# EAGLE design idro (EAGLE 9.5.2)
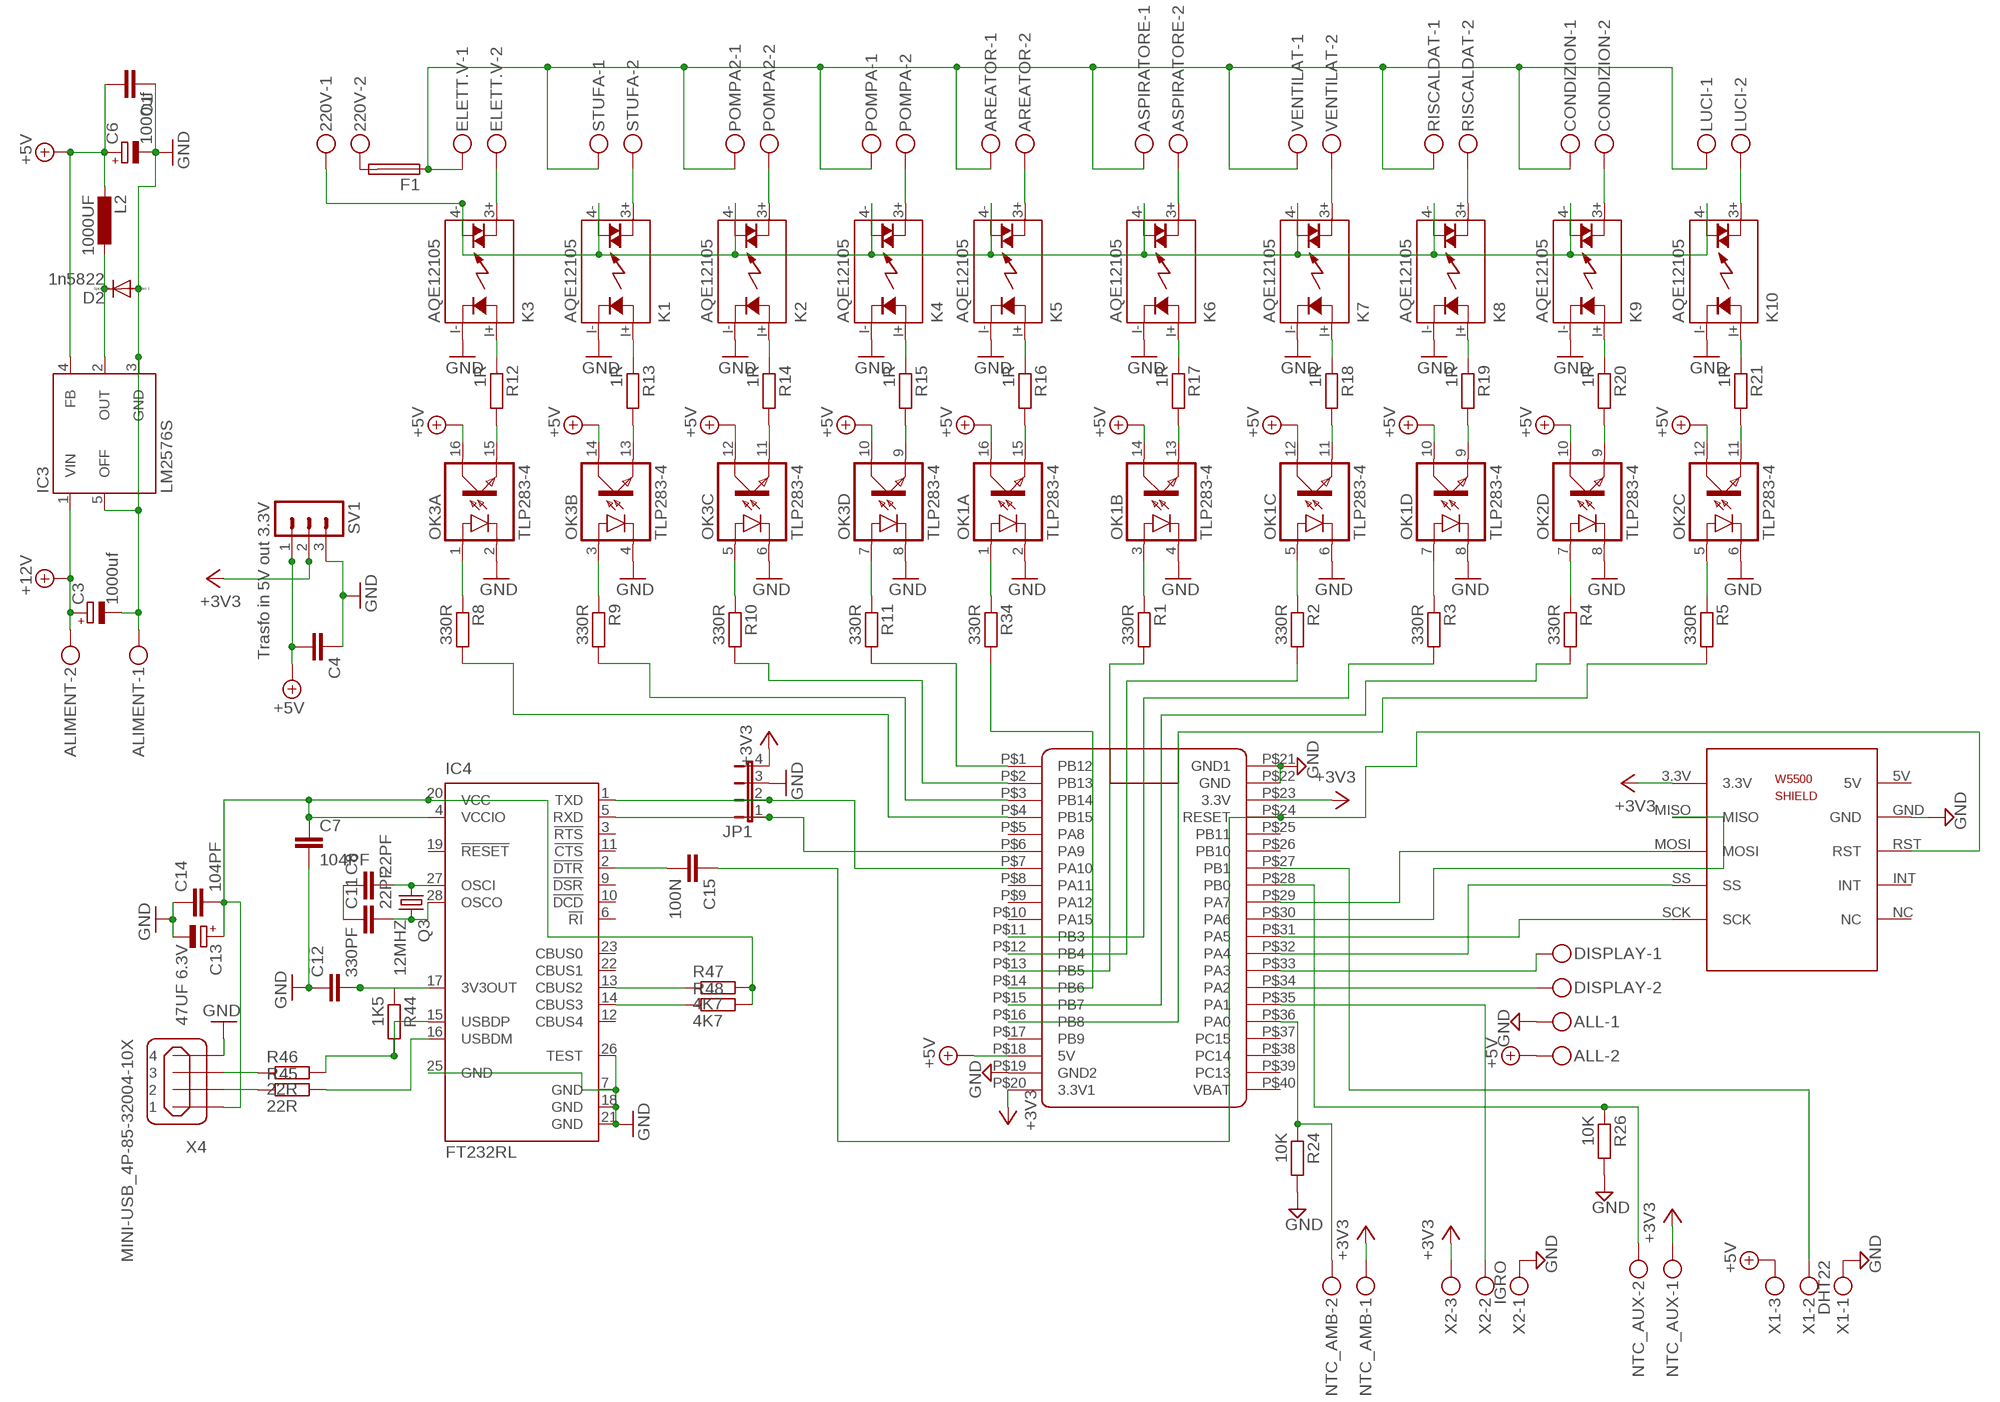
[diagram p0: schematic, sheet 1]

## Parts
220V  MKDSN1,5/2-5,08  [MKDSN1,5/2-5,08]
ALIMENT  MKDSN1,5/2-5,08  [MKDSN1,5/2-5,08]
ALL  MKDSN1,5/2-5,08  [MKDSN1,5/2-5,08]
AREATOR  MKDSN1,5/2-5,08  [MKDSN1,5/2-5,08]
ASPIRATORE  MKDSN1,5/2-5,08  [MKDSN1,5/2-5,08]
C1  C-EU025-025X050  [C025-025X050]
C3  1000uf  CPOL-EUE5-10.5  [E5-10,5]
C4  C-EU025-025X050  [C025-025X050]
C6  1000uf  CPOL-EUE5-10.5  [E5-10,5]
C7  104PF  C-EUC1206K  [C1206K]
C8  22PF  C-EUC0805  [C0805]
C11  22PF  C-EUC0805  [C0805]
C12  330PF  C-EUC1206K  [C1206K]
C13  47UF 6.3V  CPOL-EUE5-6  [E5-6]
C14  104PF  C-EUC1206K  [C1206K]
C15  100N  C-EUC0805  [C0805]
CONDIZION  MKDSN1,5/2-5,08  [MKDSN1,5/2-5,08]
D2  1n5822  DIODE-DO27-15  [DO27-15]
DISPLAY  MKDSN1,5/2-5,08  [MKDSN1,5/2-5,08]
ELETT.V  MKDSN1,5/2-5,08  [MKDSN1,5/2-5,08]
F1  SH25  [SH25]
IC3  LM2576S  [TO263-5]
IC4  FT232RL  [SSOP28]
JP1  JP4E  [JP4]
K1  AQE12105  [AQE]
K2  AQE12105  [AQE]
K3  AQE12105  [AQE]
K4  AQE12105  [AQE]
K5  AQE12105  [AQE]
K6  AQE12105  [AQE]
K7  AQE12105  [AQE]
K8  AQE12105  [AQE]
K9  AQE12105  [AQE]
K10  AQE12105  [AQE]
L2  1000UF  L-EU6000-XXX-RC  [6000-XXXX-RC]
LUCI  MKDSN1,5/2-5,08  [MKDSN1,5/2-5,08]
NTC_AMB  MKDSN1,5/2-5,08  [MKDSN1,5/2-5,08]
NTC_AUX  MKDSN1,5/2-5,08  [MKDSN1,5/2-5,08]
OK1  TLP283-4  [MINI-FLAT-16]
OK2  TLP283-4  [MINI-FLAT-16]
OK3  TLP283-4  [MINI-FLAT-16]
POMPA  MKDSN1,5/2-5,08  [MKDSN1,5/2-5,08]
POMPA2  MKDSN1,5/2-5,08  [MKDSN1,5/2-5,08]
Q3  12MHZ  CRYSTALHC49U-V  [HC49U-V]
R1  330R  R-EU_M0805  [M0805]
R2  330R  R-EU_M0805  [M0805]
R3  330R  R-EU_M0805  [M0805]
R4  330R  R-EU_M0805  [M0805]
R5  330R  R-EU_M0805  [M0805]
R8  330R  R-EU_M0805  [M0805]
R9  330R  R-EU_M0805  [M0805]
R10  330R  R-EU_M0805  [M0805]
R11  330R  R-EU_M0805  [M0805]
R12  1R  R-EU_M0805  [M0805]
R13  1R  R-EU_M0805  [M0805]
R14  1R  R-EU_M0805  [M0805]
R15  1R  R-EU_M0805  [M0805]
R16  1R  R-EU_M0805  [M0805]
R17  1R  R-EU_M0805  [M0805]
R18  1R  R-EU_M0805  [M0805]
R19  1R  R-EU_M0805  [M0805]
R20  1R  R-EU_M0805  [M0805]
R21  1R  R-EU_M0805  [M0805]
R24  10K  R-EU_M0805  [M0805]
R26  10K  R-EU_M0805  [M0805]
R34  330R  R-EU_M0805  [M0805]
R44  1K5  R-EU_M0805  [M0805]
R45  22R  R-EU_M0805  [M0805]
R46  22R  R-EU_M0805  [M0805]
R47  4K7  R-EU_M0805  [M0805]
R48  4K7  R-EU_M0805  [M0805]
RISCALDAT  MKDSN1,5/2-5,08  [MKDSN1,5/2-5,08]
STUFA  MKDSN1,5/2-5,08  [MKDSN1,5/2-5,08]
SV1  Trasfo in 5V out 3.3V  MA03-1  [MA03-1]
U$1  BLUE_PILL  [BLUE_PILL]
U$2  W5500_SHIELD  [W5500_SHIELD]
VENTILAT  MKDSN1,5/2-5,08  [MKDSN1,5/2-5,08]
X1  DHT22  MKDSN1,5/3-5,08  [MKDSN1,5/3-5,08]
X2  IGRO  MKDSN1,5/3-5,08  [MKDSN1,5/3-5,08]
X4  MINI-USB_4P-85-32004-10X  [85-32004-10X]

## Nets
+3V3: JP1.4 NTC_AMB.1 NTC_AUX.1 SV1.2 U$1.P$20(3.3V1) U$1.P$23(3.3V) U$2.3.3V X2.3
+5V: ALL.2 C1.2 C4.2 C6.+ IC3.4(FB) L2.2 OK1.10(D:COL) OK1.12(C:COL) OK1.14(B:COL) OK1.16(A:COL) OK2.10(D:COL) OK2.12(C:COL) OK3.10(D:COL) OK3.12(C:COL) OK3.14(B:COL) OK3.16(A:COL) SV1.1 U$1.P$18(5V) X1.3
+12V: ALIMENT.2 C3.+ IC3.1(VIN)
GND: ALIMENT.1 ALL.1 C1.1 C3.- C4.1 C6.- C7.2 C12.1 C13.- C14.1 D2.A IC3.3(GND) IC3.5(OFF) IC4.7(GND) IC4.18(GND) IC4.21(GND) IC4.25(GND) IC4.26(TEST) JP1.3 K1.I-(K) K2.I-(K) K3.I-(K) K4.I-(K) K5.I-(K) K6.I-(K) K7.I-(K) K8.I-(K) K9.I-(K) K10.I-(K) OK1.2(A:C) OK1.4(B:C) OK1.6(C:C) OK1.8(D:C) OK2.6(C:C) OK2.8(D:C) OK3.2(A:C) OK3.4(B:C) OK3.6(C:C) OK3.8(D:C) R24.2 R26.2 SV1.3 U$1.P$19(GND2) U$1.P$21(GND1) U$1.P$22(GND) U$2.GND X1.1 X2.1 X4.4
N$1: DISPLAY.2 U$1.P$34(PA2)
N$2: DISPLAY.1 U$1.P$33(PA3)
N$3: U$1.P$32(PA4) U$2.SS
N$5: U$1.P$31(PA5) U$2.SCK
N$6: U$1.P$29(PA7) U$2.MOSI
N$7: OK1.1(A:A) R34.1
N$8: OK1.3(B:A) R1.1
N$9: OK1.5(C:A) R2.1
N$10: OK1.7(D:A) R3.1
N$11: R34.2 U$1.P$14(PB6)
N$12: R1.2 U$1.P$13(PB5)
N$13: R2.2 U$1.P$12(PB4)
N$14: R3.2 U$1.P$11(PB3)
N$15: R4.2 U$1.P$15(PB7)
N$16: R5.2 U$1.P$16(PB8)
N$18: U$1.P$30(PA6) U$2.MISO
N$19: OK2.9(D:EMIT) R20.2
N$20: OK2.11(C:EMIT) R21.2
N$23: R11.2 U$1.P$1(PB12)
N$24: R10.2 U$1.P$2(PB13)
N$25: R9.2 U$1.P$3(PB14)
N$26: R8.2 U$1.P$4(PB15)
N$27: OK3.1(A:A) R8.1
N$28: OK3.3(B:A) R9.1
N$29: OK3.5(C:A) R10.1
N$30: OK3.7(D:A) R11.1
N$31: OK3.15(A:EMIT) R12.2
N$32: K3.I+(A) R12.1
N$33: ELETT.V.2 K3.3+(DS1)
N$34: OK3.13(B:EMIT) R13.2
N$35: K1.I+(A) R13.1
N$36: K1.3+(DS1) STUFA.2
N$37: OK3.11(C:EMIT) R14.2
N$38: K2.I+(A) R14.1
N$39: K2.3+(DS1) POMPA2.2
N$40: OK3.9(D:EMIT) R15.2
N$41: K4.I+(A) R15.1
N$42: K4.3+(DS1) POMPA.2
N$43: OK1.15(A:EMIT) R16.2
N$44: K5.I+(A) R16.1
N$45: AREATOR.2 K5.3+(DS1)
N$46: OK1.13(B:EMIT) R17.2
N$47: K6.I+(A) R17.1
N$48: ASPIRATORE.2 K6.3+(DS1)
N$49: OK1.11(C:EMIT) R18.2
N$50: K7.I+(A) R18.1
N$51: K7.3+(DS1) VENTILAT.2
N$52: OK1.9(D:EMIT) R19.2
N$53: K8.I+(A) R19.1
N$54: K8.3+(DS1) RISCALDAT.2
N$56: K9.I+(A) R20.1
N$57: CONDIZION.2 K9.3+(DS1)
N$59: K10.I+(A) R21.1
N$60: K10.3+(DS1) LUCI.2
N$61: OK2.5(C:A) R5.1
N$64: OK2.7(D:A) R4.1
N$67: 220V.2 F1.2
N$68: AREATOR.1 ASPIRATORE.1 CONDIZION.1 ELETT.V.1 F1.1 LUCI.1 POMPA2.1 POMPA.1 RISCALDAT.1 STUFA.1 VENTILAT.1
N$69: NTC_AMB.2 R24.1 U$1.P$36(PA0)
N$70: 220V.1 K1.4-(DS2) K2.4-(DS2) K3.4-(DS2) K4.4-(DS2) K5.4-(DS2) K6.4-(DS2) K7.4-(DS2) K8.4-(DS2) K9.4-(DS2) K10.4-(DS2)
N$71: U$1.P$35(PA1) X2.2
N$72: NTC_AUX.2 R26.1 U$1.P$28(PB0)
N$73: U$1.P$27(PB1) X1.2
N$77: C15.1 U$1.P$24(RESET) U$2.RST
N$95: IC4.1(TXD) JP1.2 U$1.P$7(PA10)
N$101: C7.1 C13.+ C14.2 IC4.4(VCCIO) IC4.20(VCC) R47.2 R48.2 X4.1
N$102: R45.1 X4.2
N$103: C8.2 IC4.27(OSCI) Q3.1
N$104: C11.2 IC4.28(OSCO) Q3.2
N$105: C8.1 C11.1
N$109: IC4.5(RXD) JP1.1 U$1.P$6(PA9)
N$112: D2.C IC3.2(OUT) L2.1
N$114: C12.2 IC4.17(3V3OUT) R44.1
N$124: R46.1 X4.3
N$125: IC4.15(USBDP) R44.2 R46.2
N$127: IC4.16(USBDM) R45.2
N$130: C15.2 IC4.2(!DTR)
N$131: IC4.14(CBUS3) R48.1
N$132: IC4.13(CBUS2) R47.1
Unconnected: IC4.3(!RTS) IC4.6(!RI) IC4.9(!DSR) IC4.10(!DCD) IC4.11(!CTS) IC4.12(CBUS4) IC4.19(!RESET) IC4.22(CBUS1) IC4.23(CBUS0) OK2.1(A:A) OK2.2(A:C) OK2.3(B:A) OK2.4(B:C) OK2.13(B:EMIT) OK2.14(B:COL) OK2.15(A:EMIT) OK2.16(A:COL) U$1.P$5(PA8) U$1.P$8(PA11) U$1.P$9(PA12) U$1.P$10(PA15) U$1.P$17(PB9) U$1.P$25(PB11) U$1.P$26(PB10) U$1.P$37(PC15) U$1.P$38(PC14) U$1.P$39(PC13) U$1.P$40(VBAT) U$2.5V U$2.INT U$2.NC

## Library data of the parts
220V ALIMENT ALL AREATOR ASPIRATORE CONDIZION DISPLAY ELETT.V LUCI NTC_AMB NTC_AUX POMPA POMPA2 RISCALDAT STUFA VENTILAT = con-phoenix-508:MKDSN1,5/2-5,08: MKDSN 1,5/ 2-5,08 Printklemme
C1 C4 = rcl:C-EU: CAPACITOR, European symbol
C3 C6 C13 = rcl:CPOL-EU: POLARIZED CAPACITOR, European symbol; SPICEPREFIX: C
C7 C8 C11 C12 C14 = rcl:C-EU: CAPACITOR, European symbol; SPICEPREFIX: C
C15 = resistor:C-EU: CAPACITOR, European symbol
D2 = diode:DIODE-: DIODE
F1 = fuse:SH25: FUSE HOLDER; MF: SCHURTER; MPN: 0031.8211; OC_FARNELL: 1162741; OC_NEWARK: 96B9380
IC3 = v-reg-3:LM2576: National Semiconductor 3.0A "Simple Switcher"(c) 52kHz, Vout 1.23-37V (HV: 57V), Vin 40V (HV: 60V), 50µA standby current
IC4 = ftdichip:FT232R: Source: http://www.ftdichip.com/Documents/DataSheets/DS_FT232R_v104.pdf; MPN: FT232RL; OC_FARNELL: 1146032; OC_NEWARK: 91K9918
JP1 = jumper:JP4E: JUMPER
K1-K10 = relay3:AQE*: SOLID STATE RELAY NAiS Source: http://www.mew-europe.com/.. en_ds_61610_0000.pdf; OC_FARNELL: unknown; OC_NEWARK: unknown
L2 = rcl:L-EU: INDUCTOR, European symbol; SPICEPREFIX: L
OK1-OK3 = optocoupler:TLP283-4: TOSHIBA PHOTOCOUPLER GaAs IRED & PHOTO-TRANSISTOR Source: http://www.semicon.toshiba.co.jp/td/en/Opto/Photocoupler/en_20050928_TLP283_datasheet.pdf; OC_FARNELL: unknown; OC_NEWARK: unknown
Q3 = crystal:CRYSTAL: CRYSTAL; OC_FARNELL: 1666969; OC_NEWARK: unknown
R1-R5 R8-R21 R24 R26 R34 R44-R48 = rcl:R-EU_: RESISTOR, European symbol; SPICEPREFIX: R
SV1 = con-lstb:MA03-1: PIN HEADER; OC_FARNELL: unknown; OC_NEWARK: unknown
U$1 = BluePill:BLUE_PILL
U$2 = W5500_SHIELD:W5500_SHIELD
X1 X2 = con-phoenix-508:MKDSN1,5/3-5,08: MKDSN 1,5/ 3-5,08 Printklemme Nennstrom: 13,5 A Nennspannung: 250 V Rastermaß: 5,08 mm Polzahl: 3 Anschlussart: Schraubanschluss Montage: Löten Anschlussrichtung Leiter/Platine: 0 ° Artikelnummer: 1729131 Source: http://eshop.phoenixcontact.com .. 1729131.pdf
X4 = con-cypressindustries:MINI-USB_4P-: MINI USB 4 Pol. Source: www.cypressindustries.com; OC_FARNELL: unknown; OC_NEWARK: unknown

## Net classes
0 default: width 0.203 mm, drill 0.406 mm, clearance 0.203 mm

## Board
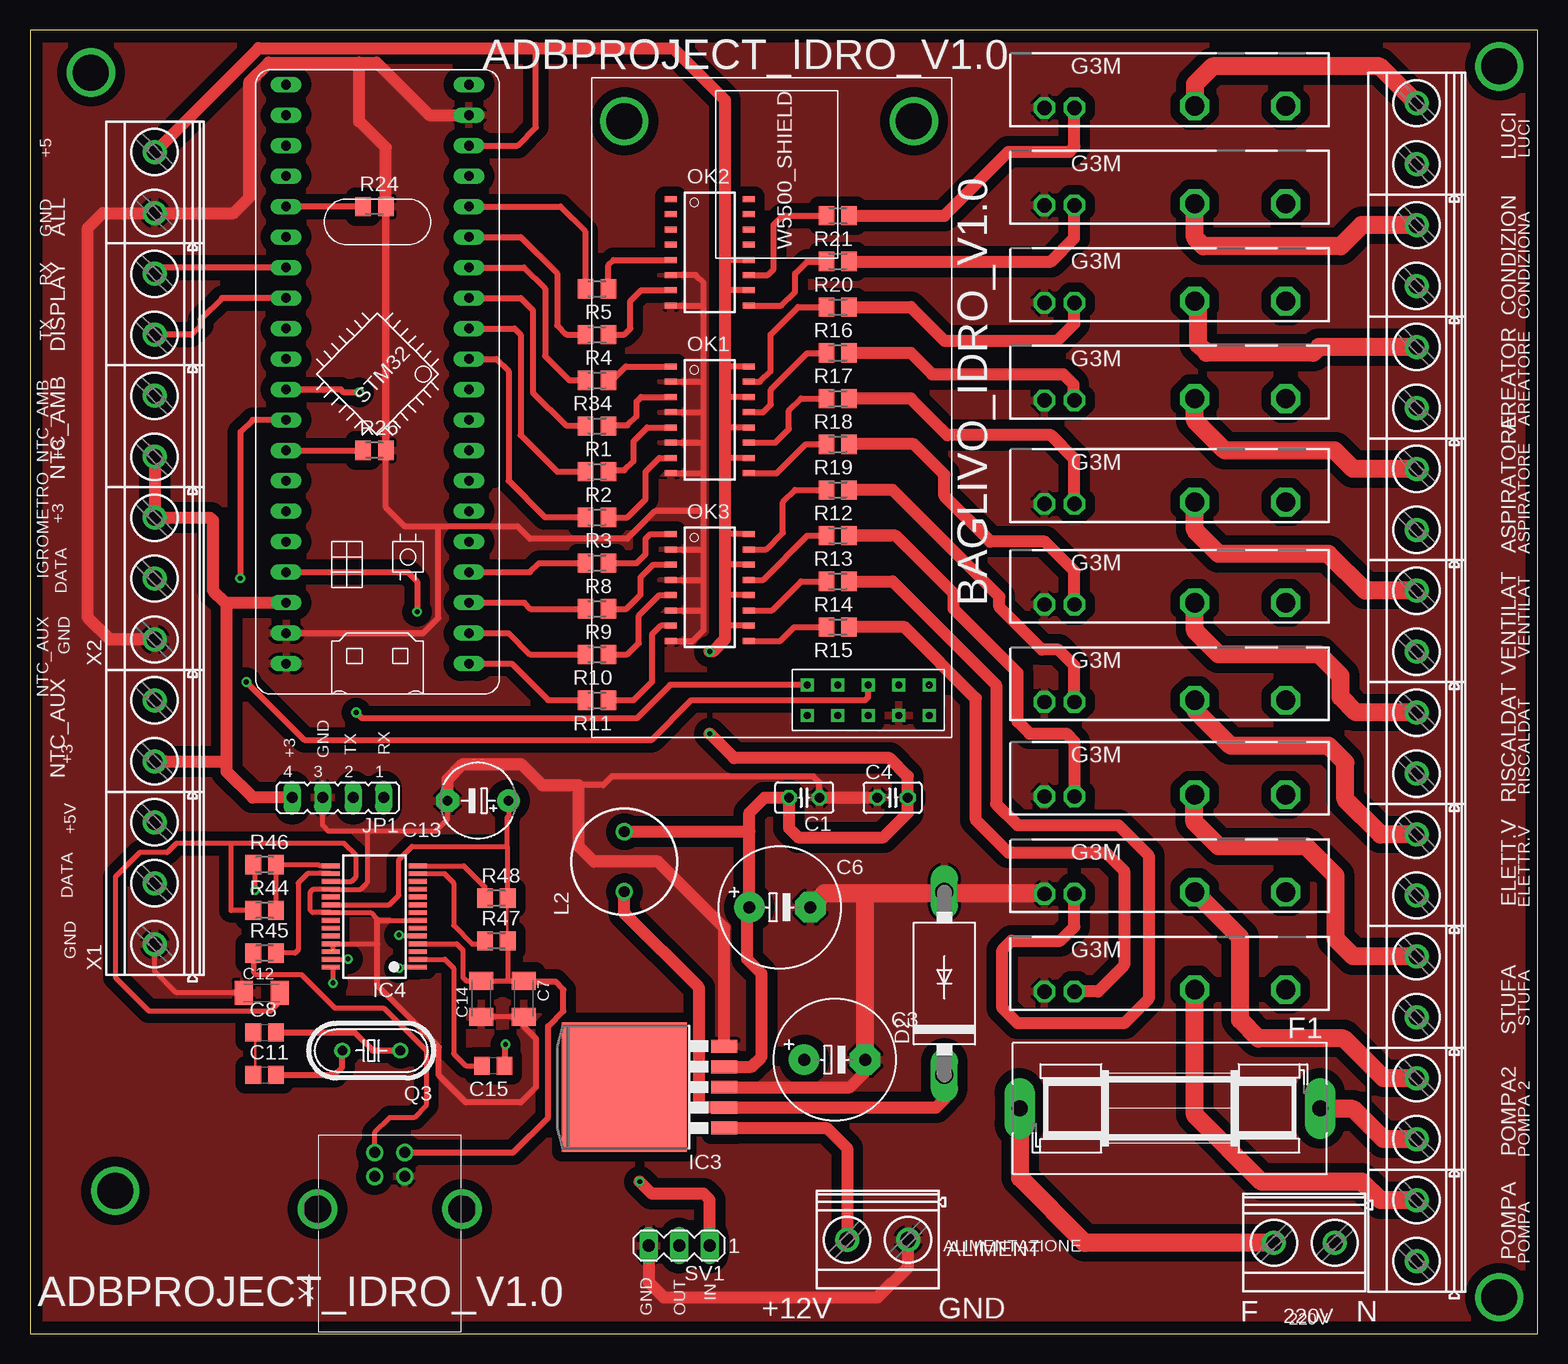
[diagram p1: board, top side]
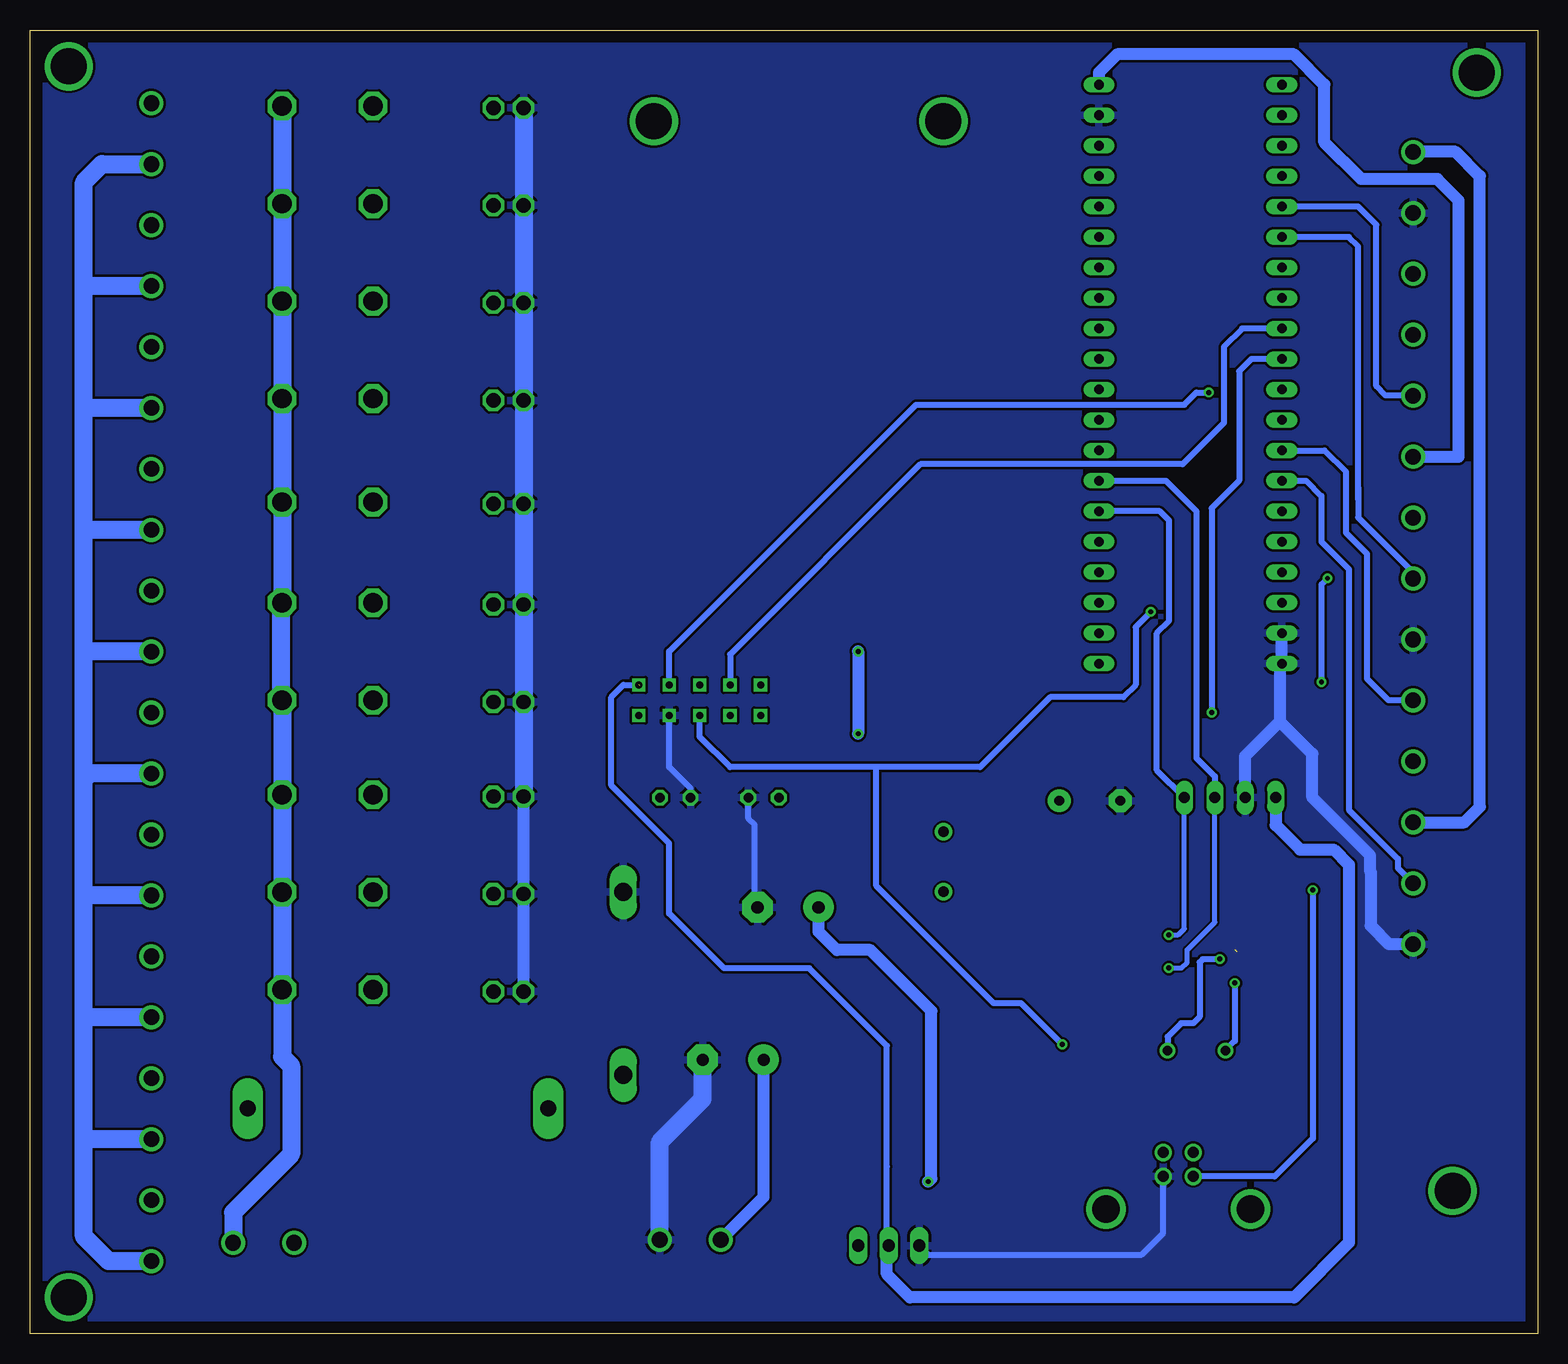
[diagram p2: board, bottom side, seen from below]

Size 125.65 x 108.7 mm. Coordinates in mm from the lower left corner, seen from the top.
Outline: 0,0 125.65,0 125.65,108.7 0,108.7 0,0
Copper layers (1*16): Top 0.035mm / dielectric 1.5mm / Bottom 0.035mm
Design rules "default": minimum track width 6mil, minimum drill 0.35mm, track to track 6mil, track to pad 6mil, pad to pad 6mil, via to via 6mil, smd to smd 6mil, copper to edge 40mil, drill to drill 6mil, minimum pad ring 10mil, minimum via ring 8mil, stop-mask expansion 4mil, vias tented up to drill 0mil, thermal gap 10mil

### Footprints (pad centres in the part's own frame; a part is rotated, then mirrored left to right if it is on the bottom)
MKDSN1,5/2-5,08 = drill 1.3 pad 2: 1 -2.561,0.025; 2 2.519,0.025
C025-025X050 = drill 0.813 octagon: 1 -1.27,0; 2 1.27,0
E5-10,5 = drill 1.016 pad 2.54: + -2.54,0 | drill 1.016 pad 2.54 octagon: - 2.54,0
C1206K = smd 1.5 x 2: 1 -1.5,0; 2 1.5,0
C0805 = smd 1.3 x 1.5: 1 -0.95,0; 2 0.95,0
E5-6 = drill 0.813 pad 1.905: + -2.54,0 | drill 0.813 pad 1.905 octagon: - 2.54,0
DO27-15 = drill 1.499 long: A 7.62,0; C -7.62,0
SH25 = drill 1.321 pad 2.54 long: 1 -12.522,0; 2 12.522,0
TO263-5 = smd 1.067 x 2.159: 1 -3.404,-5.791; 2 -1.702,-5.791; 3 0,-5.791; 4 1.702,-5.791; 5 3.404,-5.791 | smd 10.8 x 10.41: 6 0,2.54
SSOP28 = smd 0.4 x 1.5: 1 -4.225,-3.625; 2 -3.575,-3.625; 3 -2.925,-3.625; 4 -2.275,-3.625; 5 -1.625,-3.625; 6 -0.975,-3.625; 7 -0.325,-3.625; 8 0.325,-3.625; 9 0.975,-3.625; 10 1.625,-3.625; 11 2.275,-3.625; 12 2.925,-3.625; 13 3.575,-3.625; 14 4.225,-3.625; 15 4.225,3.625; 16 3.575,3.625; 17 2.925,3.625; 18 2.275,3.625; 19 1.625,3.625; 20 0.975,3.625; 21 0.325,3.625; 22 -0.325,3.625; 23 -0.975,3.625; 24 -1.625,3.625; 25 -2.275,3.625; 26 -2.925,3.625; 27 -3.575,3.625; 28 -4.225,3.625
JP4 = drill 0.914 long: 1 -3.81,0; 2 -1.27,0; 3 1.27,0; 4 3.81,0
AQE = drill 1.6 octagon: 3+ 4.612,-0.762; 4- 12.192,-0.762 | drill 1.2 octagon: I+ -5.418,-0.914; I- -7.928,-0.914
6000-XXXX-RC = drill 0.9 pad 1.422: 1 -2.5,0; 2 2.5,0
MINI-FLAT-16 = smd 1 x 0.5: 1 -3.24,4.445; 2 -3.24,3.175; 3 -3.24,1.905; 4 -3.24,0.635; 5 -3.24,-0.635; 6 -3.24,-1.905; 7 -3.24,-3.175; 8 -3.24,-4.445; 9 3.24,-4.445; 10 3.24,-3.175; 11 3.24,-1.905; 12 3.24,-0.635; 13 3.24,0.635; 14 3.24,1.905; 15 3.24,3.175; 16 3.24,4.445
HC49U-V = drill 0.813: 1 -2.413,0; 2 2.413,0
M0805 = smd 1.3 x 1.6: 1 -0.95,0; 2 0.95,0
MA03-1 = drill 1.016 long: 1 -2.54,0; 2 0,0; 3 2.54,0
BLUE_PILL = drill 0.8 long: P$1 -7.62,15.24; P$2 -7.62,12.7; P$3 -7.62,10.16; P$4 -7.62,7.62; P$5 -7.62,5.08; P$6 -7.62,2.54; P$7 -7.62,0; P$8 -7.62,-2.54; P$9 -7.62,-5.08; P$10 -7.62,-7.62; P$11 -7.62,-10.16; P$12 -7.62,-12.7; P$13 -7.62,-15.24; P$14 -7.62,-17.78; P$15 -7.62,-20.32; P$16 -7.62,-22.86; P$17 -7.62,-25.4; P$18 -7.62,-27.94; P$19 -7.62,-30.48; P$20 -7.62,-33.02; P$21 7.62,15.24; P$22 7.62,12.7; P$23 7.62,10.16; P$24 7.62,7.62; P$25 7.62,5.08; P$26 7.62,2.54; P$27 7.62,0; P$28 7.62,-2.54; P$29 7.62,-5.08; P$30 7.62,-7.62; P$31 7.62,-10.16; P$32 7.62,-12.7; P$33 7.62,-15.24; P$34 7.62,-17.78; P$35 7.62,-20.32; P$36 7.62,-22.86; P$37 7.62,-25.4; P$38 7.62,-27.94; P$39 7.62,-30.48; P$40 7.62,-33.02
W5500_SHIELD = drill 0.6 square: 3.3V 21.59,13.97; 5V 24.13,13.97; GND 24.13,11.43; INT 24.13,6.35; MISO 21.59,11.43; MOSI 21.59,8.89; NC 24.13,3.81; RST 24.13,8.89; SCK 21.59,3.81; SS 21.59,6.35 | drill 3: P$11 -25.4,12.7; P$12 -25.4,-11.43
MKDSN1,5/3-5,08 = drill 1.3 pad 2: 1 -7.641,0.025; 2 -2.561,0.025; 3 2.519,0.025
85-32004-10X = drill 0.92 pad 1.27: 1 4.71,-1.25; 2 4.71,1.25; 3 2.71,1.25; 4 2.71,-1.25 | drill 2.3 pad 3: M1 0,6.02; M2 0,-6.02

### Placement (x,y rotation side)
220V  106.17,7.62 180 top
ALIMENT  70.61,7.87 180 top
ALL  10.41,96.01 90 top
AREATOR  115.57,79.76 90 top
ASPIRATORE  115.57,69.6 90 top
C1  64.52,44.7 180 top
C3  67.06,22.86 0 top
C4  71.88,44.7 0 top
C6  62.48,35.56 0 top
C7  41.15,27.94 270 top
C8  19.56,25.15 0 top
C11  19.56,21.59 0 top
C12  19.3,28.45 0 top
C13  37.34,44.45 180 top
C14  37.59,27.94 90 top
C15  38.61,22.35 180 top
CONDIZION  115.57,89.92 90 top
D2  76.2,29.21 90 top
DISPLAY  10.41,85.85 90 top
ELETT.V  115.57,39.12 90 top
F1  95,18.8 180 top
IC3  52.07,20.57 90 top
IC4  28.7,34.8 90 top
JP1  25.65,44.7 180 top
K1  92.46,45.72 0 top
K2  92.46,37.59 0 top
K3  92.46,53.59 0 top
K4  92.46,29.46 0 top
K5  92.46,86.87 0 top
K6  92.46,78.74 0 top
K7  92.46,70.1 0 top
K8  92.46,61.72 0 top
K9  92.46,95 0 top
K10  92.46,103.12 0 top
L2  49.53,39.37 90 top
LUCI  115.57,100.08 90 top
NTC_AMB  10.41,75.69 90 top
NTC_AUX  10.41,50.29 90 top
OK1  56.64,76.2 0 top
OK2  56.64,90.17 0 top
OK3  56.64,62.23 0 top
POMPA  115.57,8.64 90 top
POMPA2  115.57,18.8 90 top
Q3  28.45,23.62 180 top
R1  47.24,75.69 180 top
R2  47.24,71.88 180 top
R3  47.24,68.07 180 top
R4  47.24,83.31 180 top
R5  47.24,87.12 180 top
R8  47.24,64.26 180 top
R9  47.24,60.45 180 top
R10  47.24,56.64 180 top
R11  47.24,52.83 180 top
R12  67.31,70.36 180 top
R13  67.31,66.55 180 top
R14  67.31,62.74 180 top
R15  67.31,58.93 180 top
R16  67.31,85.6 180 top
R17  67.31,81.79 180 top
R18  67.31,77.98 180 top
R19  67.31,74.17 180 top
R20  67.31,89.41 180 top
R21  67.31,93.22 180 top
R24  28.7,93.98 0 top
R26  28.7,73.66 0 top
R34  47.24,79.5 180 top
R44  19.56,35.31 0 top
R45  19.56,31.75 0 top
R46  19.56,39.12 0 top
R47  38.86,32.77 0 top
R48  38.86,36.32 0 top
RISCALDAT  115.57,49.28 90 top
STUFA  115.57,28.96 90 top
SV1  54.1,7.37 180 top
U$1  28.96,71.12 180 top
U$2  60.96,75.69 270 top
VENTILAT  115.57,59.44 90 top
X1  10.41,40.13 90 top
X2  10.41,65.53 90 top
X4  29.97,10.41 90 top

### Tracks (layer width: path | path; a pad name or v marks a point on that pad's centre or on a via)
+3V3  (1 unrouted)
  Top 0.203: 21.25,61 U$1.P$23 | 21.75,44.75 JP1.4
  Top 1: JP1.4 18.54,44.7 16.38,46.86 16.38,47.75 16.38,59.05 | NTC_AUX.1 11.28,47.73
  Top 1.016: NTC_AUX.1 16.36,47.73 16.38,47.75 | 16.26,60.96 U$1.P$23 | 16.26,60.96 15.24,61.98 15.24,67.82 15.01,68.05 X2.3 NTC_AMB.1 | 16.38,59.05 16.38,60.83 16.26,60.96
  Bottom 0.203: 54.25,15 54.25,13.97 54.25,7.5 SV1.2 | 74.75,54 U$2.3.3V | 36.5,104 U$1.P$20 | 10.25,73.25 NTC_AMB.1 | 22,44.5 JP1.4
  Bottom 0.5: SV1.2 54.25,7.51 54.25,13.97 54.25,24.02 60.71,30.48 67.82,30.48 72.39,35.05 72.39,40.89 77.22,45.72 77.22,53.09 76.2,54.1 74.89,54.1 74.85,54.05
  Bottom 1: JP1.4 21.84,42.42 19.81,40.39 17.02,40.39 15.75,39.12 15.75,7.62 20.32,3.05 52.32,3.05 54.25,4.97 54.25,7.5 | U$1.P$20 36.58,105.16 35.05,106.68 20.32,106.68 17.78,104.14 17.78,99.31 14.73,96.27 8.38,96.27 6.6,94.49 6.6,73.15 6.62,73.13 NTC_AMB.1
+5V  (via drill 0.41)
  Top 0.203: 49.75,41.75 L2.2 | 59.75,35.75 C6.+ | 59.75,61.5 OK3.12 | 59.75,64 OK3.14 59.75,64.25 | 59.75,87 OK2.10 | 59.75,89.5 OK2.12 | 59.75,75.5 OK1.12 | 59.75,78 OK1.14 | 59.75,80.5 OK1.16 59.75,80.75 | 59.75,66.75 OK3.16 | 11,98 10.5,98.5 ALL.2 | 36.5,99 U$1.P$18 | 59.75,59 OK3.10
  Top 0.5: U$1.P$18 40.64,99.06 42.16,100.58 42.16,107.19 | OK2.12 58.04,89.53 57.91,89.66 | OK2.10 58.04,87 57.91,86.87 | OK1.16 57.91,80.64 | OK1.14 58.04,78.11 57.91,77.98 | OK1.12 58.04,75.56 57.91,75.69 | OK1.10 58.04,73.03 57.91,72.9 | OK3.16 58.04,66.67 57.91,66.8 | OK3.14 58.04,64.14 57.91,64.26 | OK3.12 58.04,61.59 57.91,61.47 | OK3.10 58.04,59.05 57.91,58.93
  Top 1: ALL.2 19.04,107.19 42.16,107.19 53.6,107.19 57.91,102.87 57.91,89.66 57.91,86.87 57.91,80.64 57.91,77.98 57.91,75.69 57.91,72.9 57.91,66.8 57.91,64.26 57.91,61.47 57.91,58.93 57.91,57.91 56.9,56.9 v56.64,56.9 | v56.64,50.04 58.67,48.01 71.63,48.01 | 59.94,41.91 C6.+ 59.75,35.37 59.75,31.24 60.96,30.03 60.96,23.11 60.12,22.28 IC3.4 | 59.94,41.91 59.94,43.43 61.21,44.7 C1.2 63.25,42.16 64.01,41.4 71.12,41.4 73.15,43.43 C4.2 | L2.2 59.9,41.87 59.94,41.91 | SV1.1 56.64,11.18 56.13,11.68 51.82,11.68 v50.8,12.7
  Top 1.016: C4.2 73.15,46.48 71.63,48.01
  Bottom 1: v56.64,56.9 v56.64,50.04 | v50.8,12.7 50.55,12.95 50.55,26.92 55.63,32 58.42,32 59.94,33.53 C6.+ | X1.3 6.12,42.65 4.83,43.94 4.83,96.52 6.86,98.55 10.37,98.55 ALL.2
+12V
  Top 0.203: 57.75,17 57.85,17.15 IC3.1 | 68,7.75 ALIMENT.2
  Top 1: IC3.1 66.4,17.17 68.09,15.47 ALIMENT.2
  Bottom 0.203: 64.75,23 C3.+
  Bottom 1: ALIMENT.2 64.52,11.43 C3.+
GND  (1 unrouted)
  Top 0.203: 37.72,26.49 C14.1 | 25,37 IC4.18 | 28.96,34.5 32.25,34.5 IC4.7 | 26,32.5 25.25,32.5 IC4.25 | 34.08,23.92 33.95,24.05 | 28.02,37.52 28.14,37.64 | 34.75,44.25 C13.- | 24.5,44.5 JP1.3 | 53.5,60.25 OK3.6 | 53.5,62.75 OK3.4 53.5,63 | 53.5,65.25 OK3.2 53.5,65.5 | 54.25,88.25 53.5,88.25 OK2.6 | 53.5,85.75 OK2.8 | 53.5,74.25 OK1.6 | 53.5,76.75 OK1.4 | 53.5,79.25 OK1.2 53.5,79.5 | 53.5,71.75 OK1.8 | 29.75,93.75 R24.2 | 11,92.75 10.5,93.25 ALL.1 | 21.5,58.5 U$1.P$22 | 29.75,73.5 R26.2 | 57.75,20.75 IC3.3 | 57.75,23.75 IC3.5 | 69.5,22.75 C3.- 69.75,23 | 66,44.75 C1.1 | K2.I- 84.5,36.75 76.25,36.75 D2.A 76,36.75 69.6,36.75 66.25,36.75
  Top 0.4: 28.96,34.54 28.96,34.5 | 28.96,34.54 28.38,35.12 IC4.21 23.55,35.12 23.37,35.31 23.37,36.83 23.62,37.08 25.07,37.08 IC4.18 27.57,37.07 28.02,37.52 | 28.96,34.54 29.03,34.47 IC4.7 | IC4.25 28.95,32.52 28.96,32.51 | 25.25,32.05 25.25,32.5 | C7.2 37.77,26.44 37.72,26.49 | 28.14,37.64 28.14,41.86 28.19,41.91 | C13.- 34.8,42.93 33.78,41.91 28.19,41.91 | 28.19,41.91 24.89,41.91 24.38,42.42 JP1.3 | C12.1 12.19,28.45 10.39,30.25 X1.1
  Top 0.5: OK3.8 55.24,57.78 56.13,58.67 56.13,60.45 | 56.13,60.45 56.13,62.99 | 56.13,62.99 56.13,65.53 | 56.13,65.53 56.13,68.58 | 56.13,68.58 56.13,71.88 | 56.13,71.88 56.13,74.42 | 56.13,74.42 56.13,76.96 | 56.13,76.96 56.13,79.5 | 56.13,79.5 56.13,85.85 | 56.13,85.85 56.13,87.63 55.5,88.27 OK2.6 | OK1.8 56.01,71.75 56.13,71.88 | OK1.6 56.01,74.3 56.13,74.42 | OK1.4 56.01,76.83 56.13,76.96 | OK1.2 56.01,79.38 56.13,79.5 | OK2.8 56.01,85.72 56.13,85.85 | OK3.6 56.01,60.33 56.13,60.45 | OK3.4 56.01,62.87 56.13,62.99 | OK3.2 56.01,65.41 56.13,65.53 | 56.13,68.58 52.07,68.58 49.78,66.29 41.66,66.29 40.64,67.31 34.04,67.31 | R26.2 29.65,73.41 29.65,68.9 31.24,67.31 34.04,67.31 | U$1.P$22 32.77,58.42 34.04,59.69 34.04,67.31 | C1.1 65.79,45.97 65.28,46.48 48.48,46.48 47.75,45.75 45.72,45.75 | C7.2 41.15,25.65 42.16,24.64 42.16,20.57 40.89,19.3 36.32,19.3 34.08,21.55 34.08,23.92 | 33.95,24.05 28.96,29.04 28.96,32.51 28.96,34.5 28.98,34.47
  Top 0.61: R24.2 29.65,73.41
  Top 1: 69.6,36.83 D2.A 76.35,36.68 K2.I- | IC3.3 68.33,20.57 69.5,21.75 69.5,22.75 | IC3.5 57.86,33.83 52.32,39.37 46.99,39.37 45.72,40.64 45.72,45.75 42.67,45.75 40.92,47.5 36.07,47.5 34.8,46.23 C13.- | C1.1 70.45,44.7 70.5,44.75 | SV1.3 51.56,4.32 52.83,3.05 70.61,3.05 73.17,5.61 ALIMENT.1 | ALL.1 17,93.45 18.29,94.74 18.29,104.39 19.88,105.98 27.43,105.98 | U$1.P$19 33.27,101.6 28.89,105.98 27.43,105.98 | R24.2 29.65,98.87 27.43,101.09 27.43,105.98
  Top 1.016: X2.1 6.62,57.89 4.83,59.69 4.83,92.2 6.08,93.45 ALL.1
  Top 1.5: 66.37,36.75 69.6,36.75 | 69.6,36.75 84.5,36.75 | C3.- 69.6,36.75 | C6.- 66.21,36.75 66.25,36.75
  Bottom 0.203: 24.25,44.75 JP1.3 | 10.5,32.67 X1.1 | K10.I- 84.5,102 84.5,94.25 K9.I- 84.5,94 84.5,86.11 84.5,86 K5.I- 84.5,85.75 84.5,78 K6.I- 84.5,77.75 84.5,69.25 K7.I- 84.5,69 84.5,68.83 84.5,61 K8.I- | 65.75,42.93 65.75,44.5 C1.1 | K1.I- 84.51,44.95 84.5,45 84.5,45.21 84.5,52.5 K3.I- 84.5,52.75
  Bottom 0.5: C4.1 70.61,45.47 72.39,47.24 U$2.GND | C6.- 65.28,35.81 65.28,42.45 65.75,42.93 65.79,42.96 C1.1 | SV1.3 50.8,6.6 33.02,6.6 31.22,8.4 X4.4
  Bottom 1: X1.1 12.42,32.49 13.95,34.02 13.95,38.58 13.97,38.61 13.97,39.88 18.8,44.7 18.8,48.35 21.5,51.05 | 21.5,51.05 21.5,55.72 U$1.P$21 U$1.P$22 | JP1.3 24.38,48.17 21.5,51.05 | K4.I- K2.I- 84.53,44.93 84.51,44.95 | 84.53,45.18 84.5,45.21
  Bottom 1.5: K10.I- 84.53,94.03 84.5,94 | K9.I- 84.53,86.13 84.5,86.11 | K5.I- 84.53,77.78 84.5,77.75 | K6.I- 84.53,68.86 84.5,68.83 | K7.I- 84.53,61.03 84.5,61 | K8.I- 84.53,52.78 84.5,52.75 | K3.I- 84.53,44.93 | ALIMENT.1 73.17,16 69.6,19.58 C3.-
  pour Top (isolate 0.813): 0.25,108.71 125.22,108.71 125.48,108.46 125.48,0.51 124.97,0 0.76,0 0.25,0.51
  pour Bottom: 0.25,108.71 125.48,108.71 125.48,0.25 125.22,0 0.76,0 0.25,0.51
N$1
  Top 0.5: U$1.P$34 10.92,88.9 DISPLAY.2
N$2
  Top 0.5: U$1.P$33 16,86.36 14.22,84.58 14.22,84.07 13.44,83.29 DISPLAY.1
N$3
  Bottom 0.5: U$2.SS 67.31,56.64 51.45,72.5 29.61,72.5 26.16,75.95 26.16,82.3 24.64,83.82 U$1.P$32
N$4  (via drill 3)
  other vias: 5.08,105.16
N$5  (via drill 0.41)
  Top 0.5: U$2.SCK 53.34,54.1 50.55,51.31 27.69,51.31 v27.18,51.82
  Bottom 0.5: U$1.P$31 23.88,81.28 24.89,80.26 24.89,71.12 27.18,68.83 v27.18,51.82
N$6  (via drill 0.41)
  Top 0.203: 69.75,54 U$2.MOSI
  Top 0.5: U$1.P$29 18.54,76.2 17.53,75.18 v17.53,62.99 | v18.03,54.36 22.86,49.53 51.82,49.53 55.12,52.83 69.59,52.83 69.85,53.09 U$2.MOSI
  Bottom 0.5: v17.53,62.99 18.03,62.48 v18.03,54.36
N$7
  Top 0.5: R34.1 48.51,79.5 49.66,80.64 OK1.1
N$8
  Top 0.5: R1.1 48.25,75.75 49.78,75.75 50.55,76.51 50.55,77.72 50.93,78.11 OK1.3
N$9
  Top 0.5: R2.1 48.31,72 49.53,72 50.29,72.76 50.29,74.42 51.44,75.56 OK1.5
N$10
  Top 0.5: R3.1 49.78,68.07 51.31,69.6 51.31,71.88 52.45,73.03 OK1.7
N$11
  Top 0.5: U$1.P$14 41.15,88.9 42.93,87.12 42.93,81.53 44.96,79.5 R34.2
N$12
  Top 0.203: 46.27,75.72 R1.2
  Top 0.5: 46.27,75.72 44.67,75.72 41.91,78.49 41.91,85.34 40.89,86.36 U$1.P$13
N$13
  Top 0.5: U$1.P$12 40.39,83.82 40.89,83.31 40.89,74.93 43.94,71.88 R2.2
N$14
  Top 0.203: 46.29,68.09 R3.2
  Top 0.5: U$1.P$11 38.86,81.28 39.88,80.26 39.88,71.12 42.91,68.09 46.29,68.09
N$15
  Top 0.203: 46.21,83.54 46.25,83.5 R4.2
  Top 0.5: U$1.P$15 40.89,91.44 43.92,88.41 43.92,84.1 44.7,83.31 45.97,83.31 46.21,83.54
N$16
  Top 0.203: 46.25,87.25 R5.2
  Top 0.5: U$1.P$16 44.2,93.98 46.25,91.93 46.25,87.25
N$17  (via drill 3)
  other vias: 7.11,11.94
N$18  (via drill 0.41)
  Top 0.5: 24.64,78.74 U$1.P$30 25.91,78.74 26.16,78.49 v27.43,78.49
  Bottom 0.203: 72.25,54.25 U$2.MISO
  Bottom 0.5: U$2.MISO 72.39,56.9 51.82,77.47 29.46,77.47 28.45,78.49 v27.43,78.49
N$19
  Top 0.5: OK2.9 62.61,85.72 63.75,86.87 63.75,88.39 64.77,89.41 R20.2
N$20
  Top 0.203: 62,88.75 61.98,88.75 | 66.25,93 R21.2
  Top 0.5: OK2.11 61.49,88.27 61.98,88.75 61.98,92.46 62.74,93.22 R21.2
N$21  (via drill 3)
  other vias: 122.43,3.05
N$22  (via drill 3)
  other vias: 122.43,105.66
N$23
  Top 0.5: U$1.P$1 40.13,55.88 43.18,52.83 R11.2
N$24
  Top 0.5: U$1.P$2 39.88,58.42 41.66,56.64 R10.2
N$25
  Top 0.5: U$1.P$3 41.19,60.96 41.7,60.45 R9.2
N$26
  Top 0.5: U$1.P$4 41.66,63.5 42.42,64.26 R8.2
N$27
  Top 0.5: R8.1 50.56,64.26 51.31,65.01 51.31,66.29 51.69,66.67 OK3.1
N$28
  Top 0.203: 50.76,61.51 50.89,61.64
  Top 0.5: R9.1 49.7,60.45 50.76,61.51 | 50.89,61.64 50.89,63.08 51.94,64.14 OK3.3
N$29
  Top 0.203: 53.25,61.5 OK3.5
  Top 0.5: R10.1 49.78,56.64 50.74,57.6 50.74,59.88 52.45,61.59 OK3.5
N$30
  Top 0.5: R11.1 50.29,52.83 51.82,54.36 51.82,58.29 52.58,59.05 OK3.7
N$31
  Top 0.5: OK3.15 61.34,65.41 62.74,66.8 62.74,69.34 63.75,70.36 R12.2
N$32
  Top 1: K3.I+ 87.04,55.71 85.69,57.06 84.33,57.06 80.77,60.61 80.77,61.47 71.88,70.36 R12.1
N$33
  Top 0.203: 109.61,47.64 109.49,47.76
  Top 1.5: ELETT.V.2 112.54,41.63 109.61,44.56 109.61,47.64 | 109.49,47.76 108.22,49.03 100.09,49.03 100.08,49.02 97.07,52.03 K3.3+
N$34
  Top 0.5: OK3.13 61.09,62.87 64.77,66.55 R13.2
N$35
  Top 0.203: 68.5,66.5 R13.1
  Top 1: 71.63,66.55 R13.1 72.14,66.55 76.96,61.72 76.96,60.45 82.3,55.12 82.3,51.05 83.31,50.04 86.36,50.04 87.04,49.36 K1.I+
N$36
  Top 1.5: STUFA.2 110.26,31.48 108.81,32.93 108.81,38.19 106.36,40.64 99.06,40.64 97.03,42.67 97.03,44.92 K1.3+
N$37
  Top 0.5: OK3.11 61.85,60.33 64.26,62.74 R14.2
N$38
  Top 0.203: 68.5,62.5 R14.1
  Top 1: K2.I+ 87.04,33.95 85.85,32.77 81.79,32.77 81.03,32 81.03,27.18 82.3,25.91 91.19,25.91 93.22,27.94 93.22,39.88 90.68,42.42 82.3,42.42 80.52,44.2 80.52,54.1 71.88,62.74 R14.1
N$39
  Top 1.5: POMPA2.2 112.8,21.32 109.47,24.64 102.36,24.64 100.84,26.16 100.84,33.06 K2.3+
N$40
  Top 0.5: OK3.9 62.53,57.78 63.67,58.93 R15.2
N$41
  Top 1: K4.I+ 89,28.55 91.19,30.73 91.19,38.61 89.66,40.13 81.53,40.13 78.83,42.83 78.83,52.99 72.9,58.93 R15.1
N$42
  Top 1.5: POMPA.2 112.54,11.15 111,12.7 102.62,12.7 97.07,18.25 K4.3+
N$43
  Top 0.5: OK1.15 60.83,79.38 61.72,80.26 61.72,83.31 64.01,85.6 R16.2
N$44
  Top 0.203: 87.02,85.87 K5.I+
  Top 1: R16.1 73.41,85.6 76.2,82.8 85.6,82.8 87.02,84.23 87.02,85.87
N$45
  Top 0.203: 97.34,85.91 97.25,86 K5.3+
  Top 1.5: AREATOR.2 107.42,82.28 106.93,81.79 98.04,81.79 97.34,82.49 97.34,85.91
N$46
  Top 0.203: 66.25,81.75 R17.2
  Top 0.5: OK1.13 61.09,76.83 61.73,77.48 61.73,78.73 64.75,81.75 66.25,81.75
N$47
  Top 0.203: 86.94,78.06 87,78 K6.I+
  Top 1: R17.1 73.41,81.79 75.18,80.01 86.11,80.01 86.94,79.17 86.94,78.06
N$48
  Top 1.5: ASPIRATORE.2 110.26,72.11 108.71,73.66 99.57,73.66 97.07,76.16 K6.3+
N$49
  Top 0.5: OK1.11 62.1,74.3 63.25,75.44 63.25,76.96 64.26,77.98 R18.2
N$50
  Top 1: K7.I+ 87.04,72.98 85.09,74.93 76.45,74.93 73.41,77.98 R18.1
N$51
  Top 1.5: VENTILAT.2 111.27,61.95 108.2,65.02 99.06,65.02 97.07,67.02 K7.3+
N$52
  Top 0.5: OK1.9 62.24,71.75 64.66,74.17 R19.2
N$53
  Top 1: K8.I+ 87.04,63.58 84.58,66.04 80.01,66.04 76.2,69.85 76.2,71.63 73.66,74.17 R19.1
N$54
  Top 1.5: RISCALDAT.2 115.52,51.82 110.49,51.82 109.22,53.09 109.22,54.86 107.44,56.64 99.06,56.64 97.07,58.63 K8.3+
N$56
  Top 0.203: 87.01,94.03 K9.I+
  Top 1: R20.1 85.09,89.41 87.01,91.33 87.01,94.03
N$57
  Top 1.5: CONDIZION.2 110.98,92.44 109.22,90.68 97.79,90.68 97.07,91.4 K9.3+
N$59
  Top 1: R21.1 76.2,93.22 81.53,98.55 86.61,98.55 87.04,98.98 K10.I+
N$60
  Top 0.203: 97.08,102.37 K10.3+
  Top 1.5: LUCI.2 112.48,105.66 98.55,105.66 97.08,104.19 97.08,102.37
N$61
  Top 0.5: R5.1 48.19,89.09 48.64,89.53 OK2.5
N$64
  Top 0.5: R4.1 49.53,83.31 50.04,83.82 50.04,86.11 50.93,87 OK2.7
N$67
  Top 0.203: 82.5,18.75 F1.2
  Top 1.5: 220V.2 87.91,7.59 82.5,13 82.5,18.75
N$68
  Top 0.203: 107.69,18.76 F1.1
  Top 1.5: POMPA2.1 112.8,16.23 110.27,18.76 107.69,18.76
  Bottom 0.203: 115.75,6.25 POMPA.1 | 115.75,16 POMPA2.1 | 115.75,26.25 STUFA.1 | 115.75,36.5 ELETT.V.1 | 115.75,46.5 RISCALDAT.1 | 115.75,56.75 VENTILAT.1 | 115.75,67 ASPIRATORE.1 | 115.75,77 AREATOR.1 | 115.75,87.25 CONDIZION.1 | 115.75,97.5 LUCI.1
  Bottom 1.5: POMPA.1 119.11,6.08 121.16,8.13 121.16,16.26 | 121.16,16.26 121.16,26.16 | 121.16,26.16 121.16,36.32 | 121.16,36.32 121.16,46.23 | 121.16,46.23 121.16,56.9 | 121.16,56.9 121.16,67.06 | 121.16,67.06 121.16,76.96 | 121.16,76.96 121.16,87.12 | 121.16,87.12 121.16,96.01 119.66,97.52 LUCI.1 | CONDIZION.1 120.92,87.36 121.16,87.12 | AREATOR.1 120.92,77.19 121.16,76.96 | ASPIRATORE.1 121.14,67.03 121.16,67.06 | VENTILAT.1 121.14,56.88 121.16,56.9 | RISCALDAT.1 120.67,46.72 121.16,46.23 | ELETT.V.1 120.92,36.55 121.16,36.32 | STUFA.1 120.63,26.39 120.65,26.42 120.9,26.42 121.16,26.16 | POMPA2.1 121.14,16.23 121.16,16.26
N$69
  Top 0.5: R24.1 U$1.P$36
  Bottom 0.5: NTC_AMB.2 10.41,78.23 12.7,78.23 13.46,78.99 13.46,92.46 14.99,93.98 U$1.P$36
N$70
  Bottom 0.203: K7.4- 104.75,69.5 104.75,77.47 104.75,77.75 K6.4- 104.75,78 104.75,85.85 104.75,86 K5.4- 104.75,86.25 104.75,94 K9.4- | 104.75,28.19 104.75,28.5 K4.4- 104.75,28.75 104.75,36.58 104.75,36.75 K2.4- 104.75,37 104.75,44.75 K1.4- 104.75,45 104.75,52.58 104.75,52.75 K3.4- 104.75,53 104.75,60.75 K8.4- | 108.5,7.75 220V.1
  Bottom 1.5: K10.4- K9.4- 104.65,85.95 104.75,85.85 | K5.4- 104.65,77.57 104.75,77.47 | K6.4- K7.4- K8.4- 104.75,60.86 104.75,52.58 | K3.4- K1.4- 104.65,36.68 104.75,36.58 | K2.4- 104.65,28.3 104.75,28.19 | K4.4- 104.65,23.11 103.89,22.35 103.89,14.99 108.73,10.14 220V.1
N$71
  Bottom 0.5: U$1.P$35 15.75,91.44 14.99,90.68 14.99,70.61 14.99,69.6
  Bottom 0.508: 14.99,70.61 14.99,68.07 10.39,63.48 X2.2
N$72
  Top 0.5: U$1.P$28 R26.1
  Bottom 0.5: U$1.P$28 17.78,73.66 16,71.88 16,66.8 14.22,65.02
  Bottom 0.508: NTC_AUX.2 12.43,52.81 14.22,54.61 14.22,65.02
N$73
  Bottom 0.5: U$1.P$27 19.3,71.12 18.03,69.85 18.03,66.04 15.75,63.75 15.75,43.69 11.66,39.6 11.66,38.84 X1.2
N$77  (via drill 0.41)
  Top 0.5: U$1.P$24 31.5,63.5 32.26,62.74 v32.26,60.2 | v39.62,24.13 39.56,24.06 C15.1
  Bottom 0.203: 69.75,50.5 69.75,51.5 U$2.RST
  Bottom 0.5: v32.26,60.2 33.53,58.93 33.53,54.1 34.54,53.09 40.64,53.09 46.48,47.24 55.12,47.24 | U$2.RST 69.85,49.78 67.31,47.24 55.12,47.24 | v39.62,24.13 43.06,27.56 45.34,27.56 55.12,37.34 55.12,47.24
N$95  (via drill 0.41)
  Top 0.4: IC4.1 30.82,30.57 v30.75,30.5
  Bottom 0.4: v30.75,30.5 29.7,30.5 29.23,30.97 29.23,32.02 26.92,34.33 JP1.2
  Bottom 0.5: U$1.P$7 30.99,71.12 28.45,68.58 28.45,48.01 26.92,46.48 JP1.2
N$101
  Top 0.203: C14.2 37.75,29.5 39.75,29.5 41,29.5 C7.1 41.2,29.35 | 27.5,35.75 25.25,35.75 IC4.20 | 39.75,36.5 R48.2 39.75,36.25 39.75,33 R47.2 | 39.75,44.25 C13.+
  Top 0.4: IC4.4 35.55,32.52 36.07,32 36.07,29.72 36.35,29.44 C14.2 41.31,29.44 41.4,29.35 | R47.2 39.81,29.56 39.75,29.5 | IC4.20 29.93,35.77 30.73,36.58 30.73,39.52 31.85,40.64 39.75,40.64 | 39.75,40.64 39.75,36.25 | C13.+ 39.88,43.18 39.75,43.05 39.75,40.64
  Top 0.5: X4.1 40.27,15.12 43.18,18.03 43.18,25.65 44.45,26.92 44.45,28.7 43.8,29.35 41.4,29.35 41.2,29.35
N$102
  Top 0.203: 18.75,30.5 18.75,31.75 R45.1 | 28.75,15.25 X4.2
  Top 0.4: R45.1 18.61,30.16 18.8,29.97 22.61,29.97 25.4,27.18 29.46,27.18 33.02,23.62 33.02,19.05 32,18.03 29.97,18.03 28.7,16.76 28.7,15.14 X4.2
N$103  (via drill 0.41)
  Top 0.203: 30.75,23.75 Q3.1
  Top 0.4: IC4.27 26.47,31.22 v26.5,31.25
  Top 0.5: C8.2 27.04,25.15 28.56,23.62 Q3.1
  Bottom 0.5: v26.5,31.25 v26.51,31.24 27.94,31.24 28.19,30.99 28.19,26.42 28.7,25.91 29.72,25.91 30.86,24.77 Q3.1
N$104  (via drill 0.41)
  Top 0.203: 26,23.5 Q3.2 | 25.25,30.5 IC4.28
  Top 0.4: v25.25,29.25 25.25,30.5
  Top 0.5: C11.2 25.4,21.59 26,22.19 26,23.5
  Bottom 0.203: 26.03,23.65 Q3.2
  Bottom 0.5: v25.25,29.25 25.25,24.43 26.03,23.65
N$105
  Top 0.203: C11.1 18.75,21.75 18.75,25 C8.1
N$109  (via drill 0.41)
  Top 0.4: IC4.5 30.83,33.17 v30.75,33.25
  Bottom 0.203: 36.5,68.5 U$1.P$6 | 29.5,44.75 JP1.1
  Bottom 0.4: v30.75,33.25 30.73,33.27 29.97,33.27 29.46,33.78 JP1.1
  Bottom 0.5: JP1.1 31.75,46.99 31.75,58.42 30.73,59.44 30.73,67.82 31.5,68.58 U$1.P$6
N$112
  Top 0.203: 55.75,19.05 55.75,19 55.88,19
  Top 1: D2.C 76.2,19.56 75.51,18.87 IC3.2 56.01,18.87 55.88,19 | 55.75,19.05 55.75,28.83 49.53,35.05 L2.1
N$114
  Top 0.203: 26,37.75 25.25,37.75 IC4.17 | 18.5,35.5 R44.1 | 20.75,28.5 C12.2
  Top 0.4: IC4.17 26.8,37.72 27.18,38.1 27.18,39.88 26.16,40.89 16.76,40.89 | 16.76,40.89 12.19,40.89 11.43,40.13 9.14,40.13 7.11,38.1 7.11,29.72 9.91,26.92 20.07,26.92 20.83,27.69 20.83,28.42 C12.2 | R44.1 16.76,35.31 16.76,40.89
N$124  (via drill 0.41)
  Top 0.4: v18.75,37 18.75,38.97 R46.1
  Bottom 0.5: v18.75,37 18.75,16.3 21.93,13.12 X4.3
N$125
  Top 0.203: 25,39 IC4.15 | 20.5,38.86 20.5,39 R46.2
  Top 0.4: R46.2 24.01,39.12 24.11,39.02 IC4.15 | R44.2 20.51,38.85 20.5,38.86
N$127
  Top 0.203: R45.2 21.5,31.75
  Top 0.4: IC4.16 23.13,38.37 22.35,37.59 22.35,32 22.1,31.75 R45.2
N$130
  Top 0.4: IC4.2 34.56,31.22 35.31,30.48 35.31,23.37 36.32,22.35 C15.2
N$131
  Top 0.4: IC4.14 36.16,39.02 37.91,37.27 R48.1
N$132
  Top 0.4: IC4.13 34.52,38.37 35.31,37.59 35.31,34.04 36.83,32.51 37.66,32.51 R47.1

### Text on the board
tPlace: ADBPROJECT_IDRO_V1.0 | +5 | LUCI | GND | RX | CONDIZIONA | TX | AREATORE | NTC_AMB | +3 | +3 | ASPIRATORE | IGROMETRO | DATA | BAGLIVO_IDRO_V1.0 | GND | VENTILAT | NTC_AUX | +3 | GND | TX | RX | +3 | RISCALDAT | +5V | DATA | ELETTR.V | GND | STUFA | POMPA 2 | ALIMENTAZIONE | POMPA | ADBPROJECT_IDRO_V1.0 | IN | GND | OUT | 220V | +12V | GND | F | N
